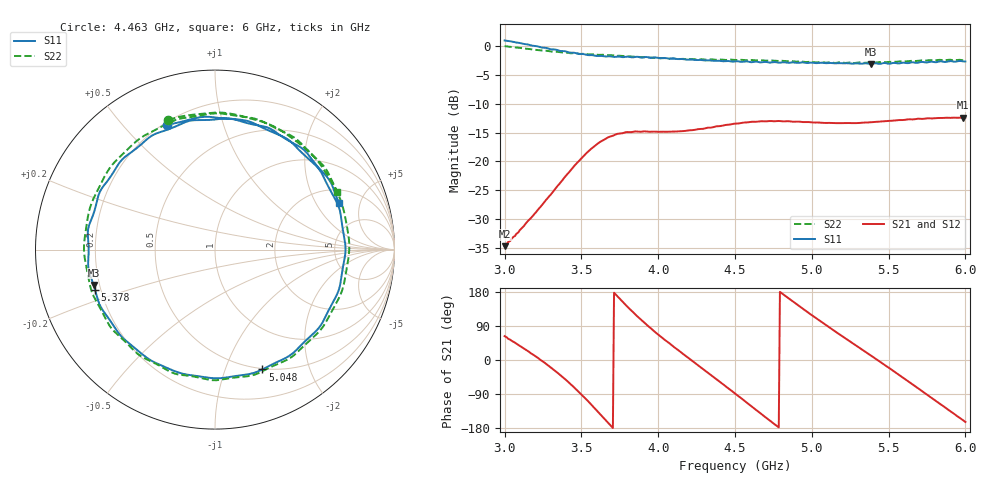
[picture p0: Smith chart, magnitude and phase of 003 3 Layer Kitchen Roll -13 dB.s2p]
!  04/11/2025  14:00:42
! Ref Plane: 0.000 mm
# MHZ S MA R  50
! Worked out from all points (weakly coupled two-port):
!   401 points, 3 GHz to 6 GHz, reference 50 ohm
!   highest |S21| = -12.39 dB at 5.985 GHz (marker M1); lowest = -34.8 dB at 3 GHz (marker M2)
!   lowest |S11| = -3.0 dB at 5.385 GHz (marker M3), VSWR 5.76, Z = 8.85 - j6.9 ohm
!   |S11| at or under -10 dB: nowhere
!   |S22| runs from -2.9 to 0.0 dB; largest |S21 - S12| = 0.006
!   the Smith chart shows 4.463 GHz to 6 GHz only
!   S11 on the Smith chart (normalised r, x): 4.463 GHz: 0.21, +0.66; 5.048 GHz: 0.49, -1.35; 5.378 GHz: 0.18, -0.16; 6 GHz: 2.82, +3.20
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3000  1.125 -115.3  0.01828 63.0  0.01841 64.2  1.006 -117.4
3270  0.9695 176.9  0.04623 -10.1  0.04612 -8.5  0.9156 174.7
3390  0.908 139.2  0.07244 -49.1  0.07267 -48.2  0.8858 136.1
3502.5  0.8576 96.6  0.1073 -92.0  0.1073 -91.1  0.8603 93.5
3600  0.8248 54.9  0.1405 -133.1  0.1409 -132.4  0.8454 53.2
3727.5  0.812 -2.9  0.1722 171.0  0.1723 172.2  0.8291 -1.5
3862.5  0.8112 -58.9  0.1816 115.7  0.1826 117.3  0.8108 -55.4
4005  0.7897 -108.8  0.1805 65.8  0.1802 66.9  0.7891 -105.0
4230  0.7647 -178.3  0.1871 -4.9  0.1871 -3.9  0.774 -176.2
4462.5  0.7434 111.3  0.2083 -76.6  0.2089 -75.3  0.7653 109.8
4500  0.7405 99.0  0.2126 -88.5  0.2137 -87.5  0.7609 98.0
4612.5  0.7289 63.7  0.2208 -123.9  0.2214 -123.0  0.7596 62.0
4755  0.7294 19.2  0.223 -168.7  0.2236 -167.6  0.7493 16.6
5002.5  0.7222 -55.1  0.2178 117.6  0.2179 118.7  0.733 -57.0
5047.5  0.7181 -68.4  0.2173 104.7  0.2177 105.7  0.7298 -70.5
5197.5  0.7119 -110.7  0.2147 63.1  0.215 64.2  0.7229 -111.4
5377.5  0.7044 -161.4  0.2181 13.8  0.2188 14.8  0.7256 -161.0
5385  0.7041 -163.8  0.2186 11.7  0.2194 12.8  0.725 -163.0
5505  0.7055 162.1  0.2248 -21.5  0.2258 -20.3  0.7334 163.4
5760  0.7288 87.9  0.2367 -94.4  0.2375 -93.2  0.757 92.0
5985  0.7394 25.2  0.2401 -158.9  0.2412 -157.8  0.7554 30.0
6000  0.7383 20.4  0.2395 -163.6  0.2402 -162.4  0.7544 25.2
